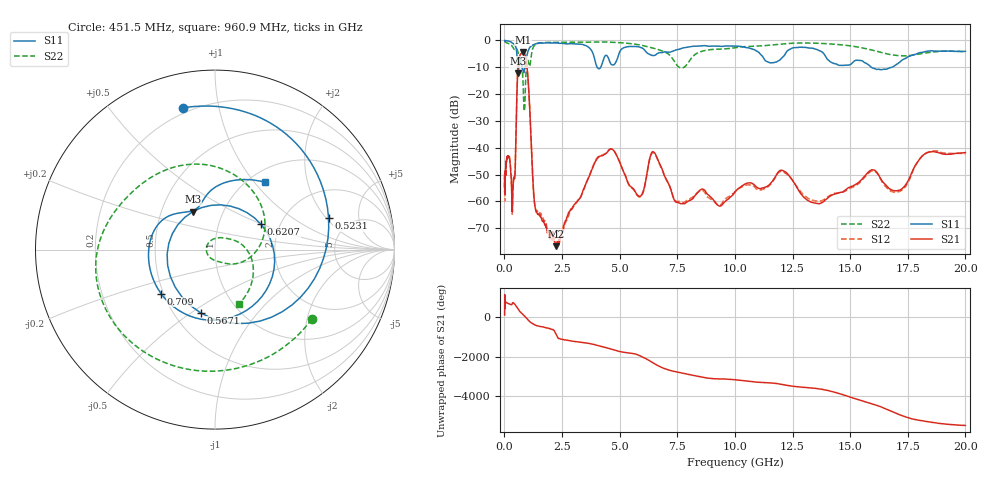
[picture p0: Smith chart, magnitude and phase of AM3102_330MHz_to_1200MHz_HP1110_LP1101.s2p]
! Date/Time: Tue, Sep 11, 2018 5:23 PM
! Network Analyzer: Agilent Technologies E8362B Rev: A.07.50.63
! Sweep from 0.010 to 20.000 GHz, 1601 Points, Sweep Type: LOG
! Power Supply: 4.949 V, 0.001 A
# Hz S DB R 50
!freq MagS11 AngS11 MagS21 AngS21 MagS12 AngS12 MagS22 AngS22
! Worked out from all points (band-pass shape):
!   1601 points, 10 MHz to 20 GHz, reference 50 ohm
!   highest |S21| = -4.30 dB at 813.7 MHz (marker M1); lowest = -76.7 dB at 2.26 GHz (marker M2)
!   |S21| within 3 dB of the highest: 614.8 MHz to 944.3 MHz (329.4 MHz wide, 42.3 % of centre)
!   lowest |S11| = -12.2 dB at 597.5 MHz (marker M3), VSWR 1.65, Z = 36 + j16.2 ohm
!   |S11| at or under -10 dB: 784.8 MHz to 893.3 MHz (108.4 MHz wide, 12.9 % of centre); 4.023 GHz to 4.18 GHz (156.5 MHz wide, 3.82 % of centre); 15.91 GHz to 16.81 GHz (897 MHz wide, 5.48 % of centre)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
!   |S22| runs from -26.3 to -0.2 dB; largest |S21 - S12| = 0.0079
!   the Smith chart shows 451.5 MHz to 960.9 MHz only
!   S11 on the Smith chart (normalised r, x): 451.5 MHz: 0.17, +0.78; 523.1 MHz: 3.42, +2.13; 567.1 MHz: 0.67, -0.55; 620.7 MHz: 1.59, +0.50; 709 MHz: 0.49, -0.28; 960.9 MHz: 1.19, +1.14
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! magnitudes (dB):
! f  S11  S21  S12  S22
! 10 MHz  0.0  -51.4  -55.1  -0.2
! 35.55 MHz  -0.1  -51.7  -51.9  -0.5
! 126.4 MHz  -0.2  -43.4  -43.6  -1.0
! 341.1 MHz  -1.0  -63.6  -64.7  -2.2
! 447.2 MHz  -1.8  -51.3  -51.1  -3.6
! 451.5 MHz  -1.8  -51.0  -50.9  -3.6
! 523.1 MHz  -3.6  -27.0  -27.1  -3.2
! 567.1 MHz  -8.8  -13.6  -13.6  -3.7
! 597.5 MHz  -12.2  -8.6  -8.7  -4.6
! 620.7 MHz  -10.7  -7.0  -7.1  -5.2
! 709 MHz  -8.2  -5.1  -5.1  -7.2
! 813.7 MHz  -11.5  -4.3  -4.4  -16.2
! 960.9 MHz  -6.6  -8.3  -8.4  -9.6
! 1.296 GHz  -1.5  -59.7  -60.1  -2.0
! 1.59 GHz  -1.0  -65.7  -64.9  -0.9
! 2.26 GHz  -1.0  -76.7  -75.0  -0.7
! 4.521 GHz  -6.7  -41.0  -40.9  -0.6
! 5.652 GHz  -2.3  -56.0  -56.3  -1.4
! 6.518 GHz  -5.6  -41.9  -42.2  -3.0
! 7.625 GHz  -3.2  -60.7  -60.0  -10.2
! 13.61 GHz  -3.6  -60.8  -59.9  -1.1
! 20 GHz  -4.1  -41.8  -42.2  -4.2
